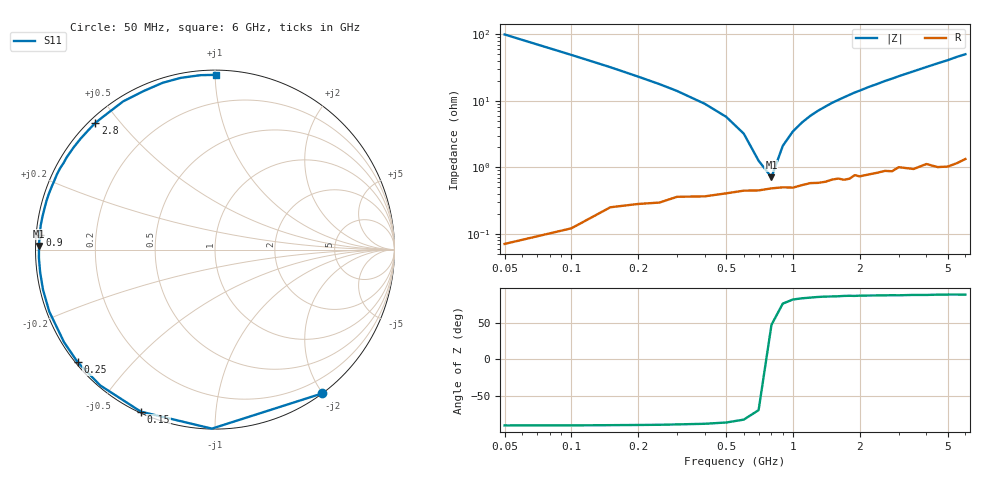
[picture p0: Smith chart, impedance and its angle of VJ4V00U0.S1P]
! Infineon Technologies  Discrete & RF Semiconductors
! BB 914
! Si Tuning Diode in SOT23
! VR = 4 V
! S-Parameters:  July  1999
# GHz  S  MA  R  50
!  f  S11
! GHz  MAG  ANG
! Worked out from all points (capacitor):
!   34 points, 50 MHz to 6 GHz, reference 50 ohm
!   read as one part to ground: C = 31.8 pF near 50 MHz
!   lowest |Z| = 713 mohm at 800 MHz (marker M1)
!   series resonance near 769.2 MHz, so ESL is about 1.3 nH
!   S11 on the Smith chart (normalised r, x): 50 MHz: 0.00, -1.99; 150 MHz: 0.01, -0.64; 250 MHz: 0.01, -0.36; 900 MHz: 0.01, +0.04; 2.8 GHz: 0.02, +0.43; 6 GHz: 0.03, +1.00
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0.05  0.9994 -53.3
0.1  0.9975 -91.0
0.15  0.9929 -114.6
0.2  0.9908 -130.2
0.25  0.9895 -140.7
0.3  0.9867 -148.5
0.4  0.9859 -159.5
0.5  0.984 -166.9
0.6  0.9823 -172.7
0.7  0.9821 -177.3
0.8  0.9808 178.8
0.9  0.9801 175.3
1  0.9804 172.1
1.2  0.9773 166.4
1.5  0.975 158.9
1.6  0.9742 156.7
1.9  0.9718 150.1
2.2  0.972 144.1
2.4  0.971 140.5
2.6  0.9698 136.6
2.8  0.9709 133.3
3  0.9675 129.7
3.5  0.9715 121.8
4  0.9687 114.3
4.5  0.974 107.4
5  0.9756 101.3
5.5  0.9751 94.8
6  0.9737 89.7
